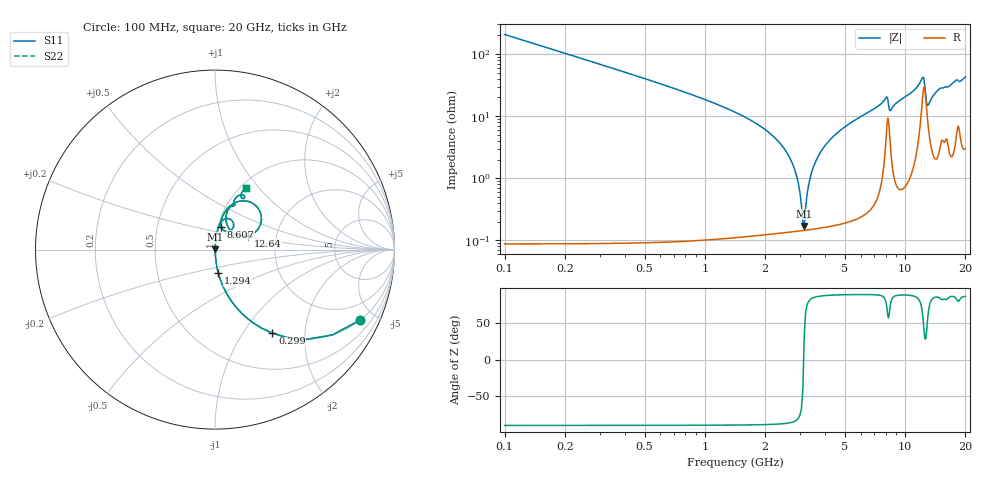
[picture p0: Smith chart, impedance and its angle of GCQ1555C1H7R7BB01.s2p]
!Murata Part Number: GCQ1555C1H7R7BB01
!These Parameters are Measured in Series Mode Connection
!Data Generated on Mar 13, 2026
!  o--ll--o
!Port1  Port2
!  o------o
!Operation Temp=25[degC], DC Bias Voltage=0[V]
!Freq. Start=100[MHz] Stop=20[GHz] 401[Steps]
# Hz S RI R 50
!Freq.(Hz) S11(Real) S11(Imag) S21(Real) S21(Imag) S12(Real) S12(Imag) S22(Real) S22(Imag)
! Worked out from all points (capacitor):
!   401 points, 100 MHz to 20 GHz, reference 50 ohm
!   read as one part in series: C = 7.7 pF near 199.5 MHz
!   lowest |Z| = 170 mohm at 3.135 GHz (marker M1)
!   series resonance near 3.114 GHz, so ESL is about 340 pH
!   S11 on the Smith chart (normalised r, x): 100 MHz: 1.00, -4.13; 299 MHz: 1.00, -1.37; 1.294 GHz: 1.00, -0.26; 8.607 GHz: 1.03, +0.27; 12.64 GHz: 1.43, +0.22; 20 GHz: 1.06, +0.85
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1e8  0.8099 -0.3922  0.1901 0.3922  0.1901 0.3922  0.8099 -0.3922
2.99e8  0.3195 -0.4656  0.6805 0.4656  0.6805 0.4656  0.3195 -0.4656
5.975e8  0.1006 -0.2994  0.8994 0.2994  0.8994 0.2994  0.1006 -0.2994
1.294e9  0.0182 -0.1297  0.9818 0.1297  0.9818 0.1297  0.0182 -0.1297
2.5875e9  0.00196 -0.0248  0.998 0.0248  0.998 0.0248  0.00196 -0.0248
2.83625e9  0.00155 -0.0125  0.9985 0.0125  0.9985 0.0125  0.00155 -0.0125
3.03525e9  0.00144 -0.00341  0.9986 0.00341  0.9986 0.00341  0.00144 -0.00341
3.13475e9  0.00145 0.000888  0.9986 -0.000888  0.9986 -0.000888  0.00145 0.000888
3.43325e9  0.00168 0.0131  0.9983 -0.0131  0.9983 -0.0131  0.00168 0.0131
3.83125e9  0.00237 0.028  0.9976 -0.028  0.9976 -0.028  0.00237 0.028
4.42825e9  0.00408 0.0484  0.9959 -0.0484  0.9959 -0.0484  0.00408 0.0484
6.7665e9  0.018 0.1205  0.982 -0.1205  0.982 -0.1205  0.018 0.1205
8.06e9  0.0802 0.1712  0.9198 -0.1712  0.9198 -0.1712  0.0802 0.1712
8.3585e9  0.0606 0.102  0.9394 -0.102  0.9394 -0.102  0.0606 0.102
8.60725e9  0.0334 0.1282  0.9666 -0.1282  0.9666 -0.1282  0.0334 0.1282
1.005e10  0.0474 0.1952  0.9526 -0.1952  0.9526 -0.1952  0.0474 0.1952
1.218925e10  0.2282 0.2442  0.7718 -0.2442  0.7718 -0.2442  0.2282 0.2442
1.2637e10  0.1827 0.0756  0.8173 -0.0756  0.8173 -0.0756  0.1827 0.0756
1.29355e10  0.0932 0.0994  0.9068 -0.0994  0.9068 -0.0994  0.0932 0.0994
1.338325e10  0.0622 0.1587  0.9378 -0.1587  0.9378 -0.1587  0.0622 0.1587
1.67165e10  0.1055 0.2704  0.8945 -0.2704  0.8945 -0.2704  0.1055 0.2704
2e10  0.1713 0.3435  0.8287 -0.3435  0.8287 -0.3435  0.1713 0.3435
